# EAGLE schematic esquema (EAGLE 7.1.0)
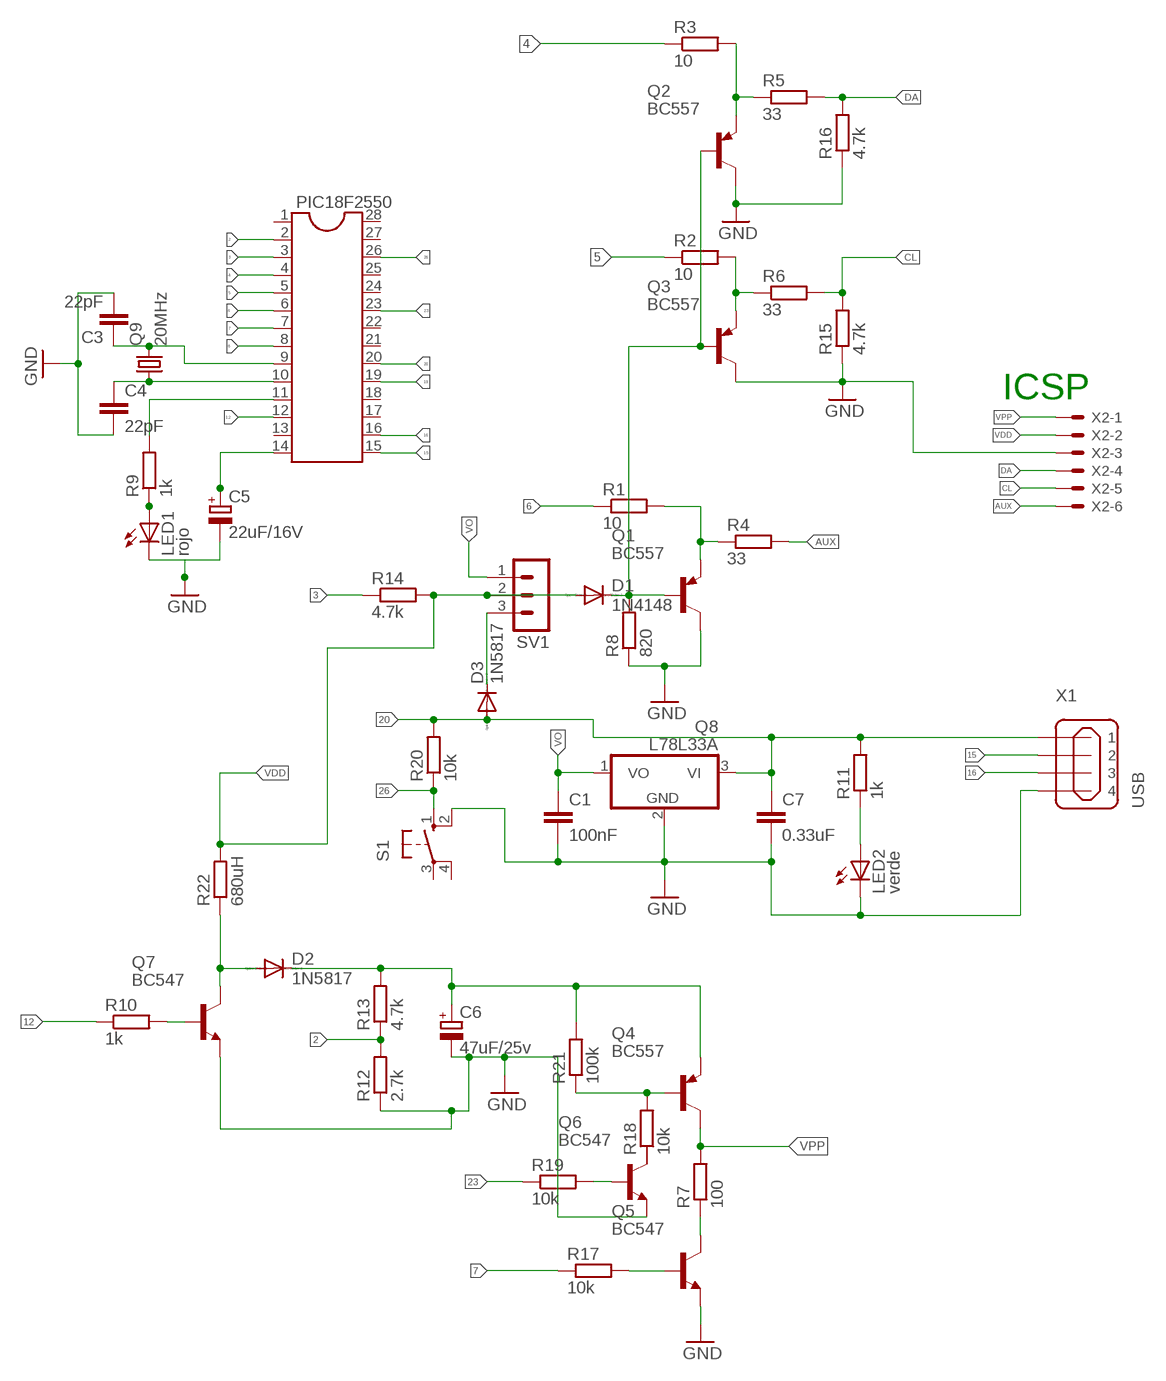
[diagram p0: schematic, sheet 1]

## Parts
C1  100nF  C-EU025-030X050  [C025-030X050]
C3  22pF  C-EU050-024X044  [C050-024X044]
C4  22pF  C-EU050-024X044  [C050-024X044]
C5  22uF/16V  CPOL-EUE2-5  [E2-5]
C6  47uF/25v  CPOL-EUE2-5  [E2-5]
C7  0.33uF  C-EU050-024X044  [C050-024X044]
D1  1N4148  1N4148DO35-7  [DO35-7]
D2  1N5817  1N4148DO35-7  [DO35-7]
D3  1N5817  1N4148DO35-7  [DO35-7]
LED1  rojo  LED3MM  [LED3MM]
LED2  verde  LED3MM  [LED3MM]
PIC18F2550  DIL28-3  [DIL28-3]
Q1  BC557  BC214  [TO92]
Q2  BC557  BC214  [TO92]
Q3  BC557  BC214  [TO92]
Q4  BC557  BC214  [TO92]
Q5  BC547  BCX59SMD  [TO92-EBC]
Q6  BC547  BCX59SMD  [TO92-EBC]
Q7  BC547  BCX59SMD  [TO92-EBC]
Q8  L78L33A  78L05Z  [TO92]
Q9  20MHz  CRYSTALHC49S  [HC49/S]
R1  10  R-EU_0207/7  [0207/7]
R2  10  R-EU_0207/7  [0207/7]
R3  10  R-EU_0207/7  [0207/7]
R4  33  R-EU_0207/7  [0207/7]
R5  33  R-EU_0207/7  [0207/7]
R6  33  R-EU_0207/7  [0207/7]
R7  100  R-EU_0207/7  [0207/7]
R8  820  R-EU_0207/7  [0207/7]
R9  1k  R-EU_0207/7  [0207/7]
R10  1k  R-EU_0207/7  [0207/7]
R11  1k  R-EU_0207/7  [0207/7]
R12  2.7k  R-EU_0207/7  [0207/7]
R13  4.7k  R-EU_0207/7  [0207/7]
R14  4.7k  R-EU_0207/7  [0207/7]
R15  4.7k  R-EU_0207/7  [0207/7]
R16  4.7k  R-EU_0207/7  [0207/7]
R17  10k  R-EU_0207/7  [0207/7]
R18  10k  R-EU_0207/7  [0207/7]
R19  10k  R-EU_0207/7  [0207/7]
R20  10k  R-EU_0207/7  [0207/7]
R21  100k  R-EU_0207/7  [0207/7]
R22  680uH  R-EU_0207/10  [0207/10]
S1  10-XX  [B3F-10XX]
SV1  MA03-1  [MA03-1]
X1  USB  MINI-USB_SHIELD4P-85-32004-00X  [85-32004-00X]
X2  22-23-2061  [22-23-2061]

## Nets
2: PIC18F2550.2 R12.2 R13.1
3: PIC18F2550.3 R14.1
4: PIC18F2550.4 R3.1
5: PIC18F2550.5 R2.1
6: PIC18F2550.6 R1.1
7: PIC18F2550.7 R17.1
8: PIC18F2550.8
11: PIC18F2550.11 R9.2
12: PIC18F2550.12 R10.1
14: C5.+ PIC18F2550.14
15: PIC18F2550.15 X1.2
16: PIC18F2550.16 X1.3
19: PIC18F2550.19
20: C7.1 D3.A PIC18F2550.20 Q8.3(VI) R11.2 R20.2 X1.1
23: PIC18F2550.23 R19.1
26: PIC18F2550.26 R20.1 S1.1(S)
AUX: R4.2 X2.6
CL: R6.2 R15.2 X2.5
DA: R5.2 R16.2 X2.4
GND: C1.2 C3.2 C4.2 C5.- C6.- C7.2 LED1.K(C) LED2.K(C) Q1.3(C) Q2.3(C) Q3.3(C) Q5.E Q6.E Q7.E Q8.2(GND) R8.1 R12.1 R15.1 R16.1 S1.2(S1) X1.4 X2.3
N$1: C3.1 PIC18F2550.9 Q9.2
N$2: C4.1 PIC18F2550.10 Q9.1
N$3: LED1.A R9.1
N$4: Q6.B R19.2
N$5: Q5.B R17.2
N$6: C6.+ D2.C Q4.1(E) R13.2 R21.2
N$7: Q5.C R7.1
N$8: Q3.1(E) R2.2 R6.1
N$9: Q4.2(B) R18.2 R21.1
N$11: Q7.B R10.2
N$12: D2.A Q7.C R22.1
N$13: D1.C Q1.2(B) Q2.2(B) Q3.2(B) R8.2
N$14: LED2.A R11.1
N$15: D3.C SV1.3
N$16: Q1.1(E) R1.2 R4.1
N$17: Q2.1(E) R3.2 R5.1
VDD: D1.A R14.2 R22.2 SV1.2 X2.2
VO: C1.1 Q8.1(VO) SV1.1
VPP: Q4.3(C) R7.2 X2.1
Unconnected: PIC18F2550.1 PIC18F2550.13 PIC18F2550.17 PIC18F2550.18 PIC18F2550.21 PIC18F2550.22 PIC18F2550.24 PIC18F2550.25 PIC18F2550.27 PIC18F2550.28 Q6.C R18.1 S1.3(P) S1.4(P1) X1.M1(S1) X1.M2(S2)

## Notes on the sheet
- ICSP

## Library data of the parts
C1 C3 C4 C7 = rcl:C-EU: CAPACITOR, European symbol
C5 C6 = rcl:CPOL-EU: POLARIZED CAPACITOR, European symbol
D1-D3 = diode:1N4148: DIODE
LED1 LED2 = led:LED: LED
PIC18F2550 = ic-package:DIL28: Dual In Line
Q1-Q4 = transistor-pnp:BC214: PNP Transistor
Q5-Q7 = transistor-npn:BCX59*: NPN Transistor
Q8 = linear:78*: Positive VOLTAGE REGULATOR Source: http://cache.national.com/ds/LM/LM78L05.pdf http://www.fairchildsemi.com/ds/LM/LM7805.pdf
Q9 = crystal:CRYSTAL: CRYSTAL; OC_FARNELL: 1667008; OC_NEWARK: unknown
R1-R22 = rcl:R-EU_: RESISTOR, European symbol
S1 = switch-omron:10-XX: OMRON SWITCH; MPN: B3F-1000; OC_FARNELL: 176432; OC_NEWARK: 36M3542
SV1 = con-lstb:MA03-1: PIN HEADER; OC_FARNELL: unknown; OC_NEWARK: unknown
X1 = con-cypressindustries:MINI-USB_SHIELD4P-: MINI USB 4 Pol. Source: www.cypressindustries.com; OC_FARNELL: unknown; OC_NEWARK: unknown
X2 = con-molex:22-23-2061: .100" (2.54mm) Center Header - 6 Pin; MF: MOLEX; MPN: 22-23-2061; OC_FARNELL: 1462922; OC_NEWARK: 27C1933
